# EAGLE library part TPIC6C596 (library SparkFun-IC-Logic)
Serial in shift register with open collector outputs This can sink up to 100mA per channel Datasheet SparkFun Products SparkFun Large Digit Driver (WIG-13279)
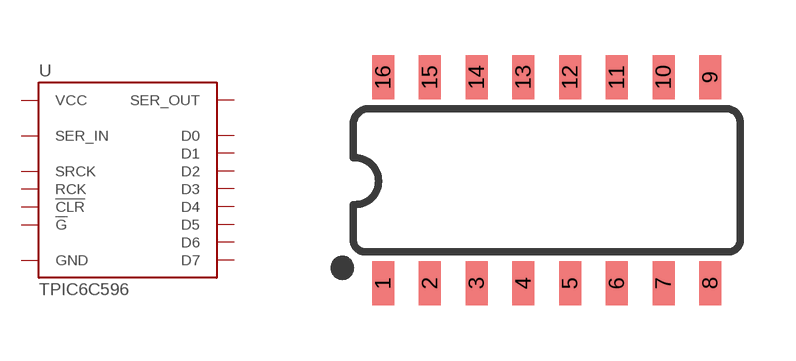
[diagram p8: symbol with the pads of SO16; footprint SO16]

Designator prefix U

## TPIC6C596SOIC (PROD_ID: IC-12522; VALUE: TPIC6C596)  [SO16]
1  VCC  pwr
2  SER_IN  in
3  D0  out
4  D1  out
5  D2  out
6  D3  out
7  !CLR  in
8  !G  in
9  SER_OUT  out
10  RCK  in
11  D4  out
12  D5  out
13  D6  out
14  D7  out
15  SRCK  in
16  GND  pwr

## Footprint SO16 (pad centres in mm)
SOIC, 0.15 inch width
smd 0.6 x 1.2: 1 -4.445,-2.8; 2 -3.175,-2.8; 3 -1.905,-2.8; 4 -0.635,-2.8; 5 0.635,-2.8; 6 1.905,-2.8; 7 3.175,-2.8; 8 4.445,-2.8; 9 4.445,2.8; 10 3.175,2.8; 11 1.905,2.8; 12 0.635,2.8; 13 -0.635,2.8; 14 -1.905,2.8; 15 -3.175,2.8; 16 -4.445,2.8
